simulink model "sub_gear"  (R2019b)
settings: Solver=VariableStepAuto  StartTime=0.0  StopTime=10.0  MaxStep=0.001  RelTol=1e-3
libraries: simulink x1

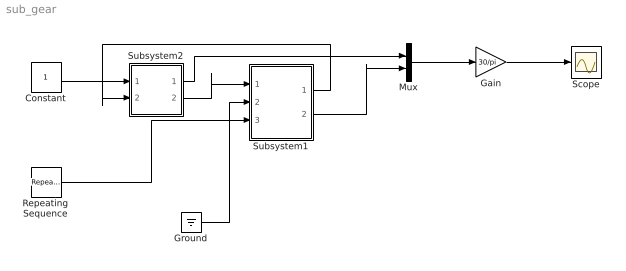
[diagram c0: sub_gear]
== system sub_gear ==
  Constant : Constant
  Gain : Gain  Gain=30/pi
  Ground : Ground
  Mux : Mux  Inputs=2
  Repeating Sequence : simulink/Sources/Repeating Sequence  rep_seq_t=[0 3 4 10]  rep_seq_y=[0 0 1 1]
  Scope : Scope
  Subsystem1 : Subsystem
  Subsystem2 : Subsystem
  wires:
  Constant/1 -> Subsystem2/1(T1)
  Subsystem2/2(w2) -> Subsystem1/1(w1)
  Repeating Sequence/1 -> Subsystem1/3(APS)
  Subsystem1/1(T1) -> Subsystem2/2(T2)
  Ground/1 -> Subsystem1/2(T2)
  Mux/1 -> Gain/1
  Gain/1 -> Scope/1
  Subsystem2/1(w1) -> Mux/1
  Subsystem1/2(w2) -> Mux/2

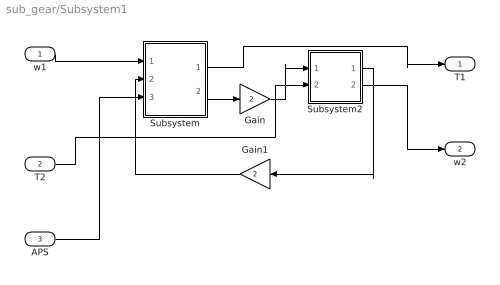
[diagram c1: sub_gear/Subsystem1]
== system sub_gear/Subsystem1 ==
  w1 : Inport
  T2 : Inport  Port=2
  APS : Inport  Port=3
  Gain : Gain  Gain=2
  Gain1 : Gain  Gain=2
  Subsystem : Subsystem
  Subsystem2 : Subsystem
  T1 : Outport
  w2 : Outport  Port=2
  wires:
  T2/1 -> Subsystem2/2(T2)
  Subsystem2/2(w2) -> w2/1
  Gain/1 -> Subsystem2/1(T1)
  Subsystem/1(T1) -> T1/1
  Gain1/1 -> Subsystem/2(w2)
  Subsystem2/1(w1) -> Gain1/1
  Subsystem/2(T2) -> Gain/1
  APS/1 -> Subsystem/3(APS)
  w1/1 -> Subsystem/1(w1)

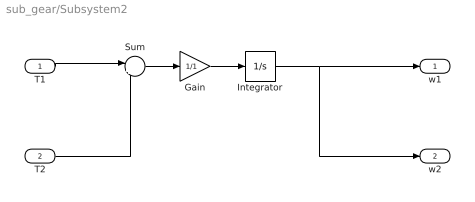
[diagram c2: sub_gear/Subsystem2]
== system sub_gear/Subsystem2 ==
  T1 : Inport
  T2 : Inport  Port=2
  Gain : Gain  Gain=1/1
  Integrator : Integrator
  Sum : Sum  Inputs=|+-
  w1 : Outport
  w2 : Outport  Port=2
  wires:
  T1/1 -> Sum/1
  Integrator/1 -> w2/1, w1/1
  T2/1 -> Sum/2
  Sum/1 -> Gain/1
  Gain/1 -> Integrator/1

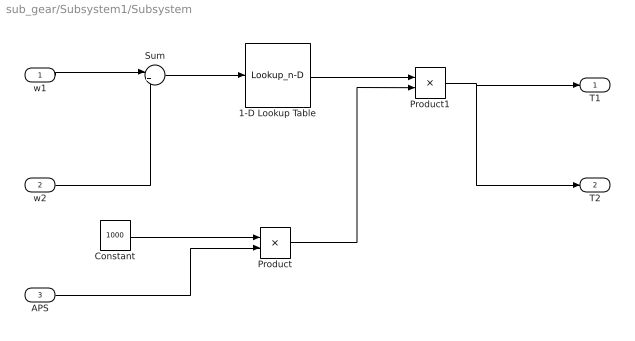
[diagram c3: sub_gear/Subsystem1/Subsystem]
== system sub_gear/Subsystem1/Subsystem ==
  w1 : Inport
  w2 : Inport  Port=2
  APS : Inport  Port=3
  1-D Lookup Table : Lookup_n-D  NumberOfTableDimensions=1  BreakpointsForDimension1=[-10:10]  Table=tanh(2*[-10:10])  InternalRulePriority=Speed  RndMeth=Simplest
  Constant : Constant  Value=1000
  Product : Product
  Product1 : Product
  Sum : Sum  Inputs=|+-
  T1 : Outport
  T2 : Outport  Port=2
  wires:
  Product1/1 -> T2/1, T1/1
  1-D Lookup Table/1 -> Product1/1
  APS/1 -> Product/2
  w2/1 -> Sum/2
  Product/1 -> Product1/2
  w1/1 -> Sum/1
  Sum/1 -> 1-D Lookup Table/1
  Constant/1 -> Product/1

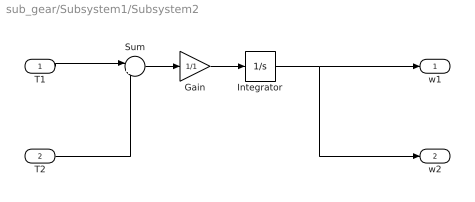
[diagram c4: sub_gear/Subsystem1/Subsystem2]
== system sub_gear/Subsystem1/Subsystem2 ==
  T1 : Inport
  T2 : Inport  Port=2
  Gain : Gain  Gain=1/1
  Integrator : Integrator
  Sum : Sum  Inputs=|+-
  w1 : Outport
  w2 : Outport  Port=2
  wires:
  T1/1 -> Sum/1
  Integrator/1 -> w2/1, w1/1
  T2/1 -> Sum/2
  Sum/1 -> Gain/1
  Gain/1 -> Integrator/1
